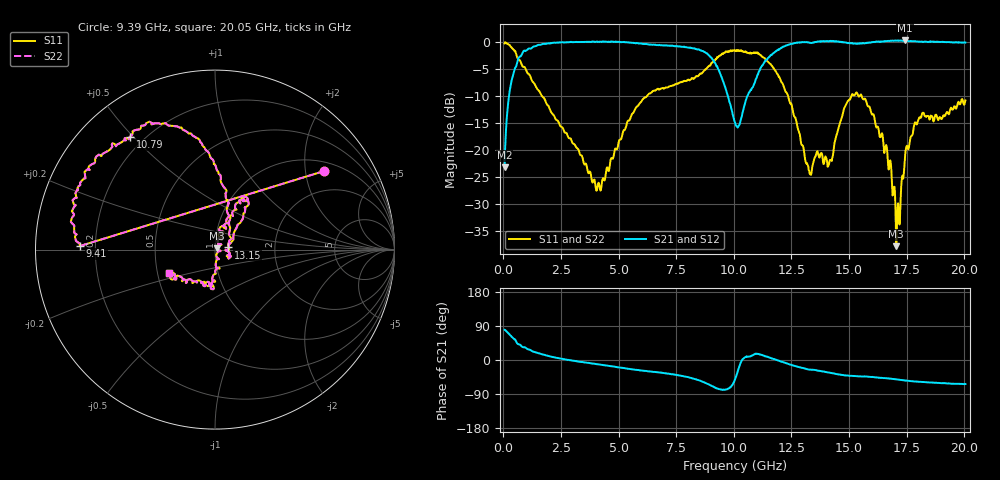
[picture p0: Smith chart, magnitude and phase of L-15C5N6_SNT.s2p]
#	mhz	s	ma	r	50
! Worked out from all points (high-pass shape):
!   1001 points, 50 MHz to 20.05 GHz, reference 50 ohm
!   highest |S21| = 0.31 dB at 17.43 GHz (marker M1); lowest = -23.2 dB at 50 MHz (marker M2)
!   |S21| within 3 dB of the highest: 708.4 MHz to 8.966 GHz (8.258 GHz wide, 171 % of centre); 11.54 GHz to end of sweep
!   lowest |S11| = -37.9 dB at 17.05 GHz (marker M3), VSWR 1.03, Z = 51.1 + j0.739 ohm
!   |S11| at or under -10 dB: 1.669 GHz to 6.236 GHz (4.567 GHz wide, 116 % of centre); 12.35 GHz to 15.1 GHz (2.748 GHz wide, 20 % of centre); 15.55 GHz to end of sweep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
!   |S22| runs from -37.9 to 0.0 dB; largest |S21 - S12| = 0
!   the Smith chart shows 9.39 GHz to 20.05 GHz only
!   S11 on the Smith chart (normalised r, x): 9.39 GHz: 1.27, +2.53; 9.41 GHz: 0.14, +0.01; 10.79 GHz: 0.15, +0.49; 13.15 GHz: 1.16, +0.03; 20.05 GHz: 0.58, -0.17
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50  0.9714 175.5  0.06904 79.7  0.06904 79.7  0.9714 175.5
310  0.9091 155.8  0.3928 64.5  0.3928 64.5  0.9091 155.8
750  0.6504 129.2  0.7373 38.7  0.7373 38.7  0.6504 129.2
1670  0.3159 100.5  0.9551 15.1  0.9551 15.1  0.3159 100.5
3390  0.08854 54.7  1.002 -5.3  1.002 -5.3  0.08854 54.7
4150  0.04844 -17.9  1.005 -11.7  1.005 -11.7  0.04844 -17.9
6730  0.3668 -115.6  0.9356 -32.7  0.9356 -32.7  0.3668 -115.6
8530  0.506 -143.6  0.8401 -54.4  0.8401 -54.4  0.506 -143.6
9390  0.7487 35.8  0.5203 -77.1  0.5203 -77.1  0.7487 35.8
9410  0.7527 178.5  0.5084 -77.5  0.5084 -77.5  0.7527 178.5
10050  0.839 153.7  0.1798 -51.3  0.1798 -51.3  0.839 153.7
10790  0.7869 126.9  0.3751 11.6  0.3751 11.6  0.7869 126.9
12070  0.4218 87.2  0.8868 -4.6  0.8868 -4.6  0.4218 87.2
13150  0.07446 9.2  1.001 -23.7  1.001 -23.7  0.07446 9.2
13390  0.06623 -3.5  0.9849 -25.5  0.9849 -25.5  0.06623 -3.5
14170  0.08047 6.2  1.02 -33.7  1.02 -33.7  0.08047 6.2
15250  0.3238 56.6  0.9695 -42.4  0.9695 -42.4  0.3238 56.6
16730  0.0656 57.0  1.027 -48.9  1.027 -48.9  0.0656 57.0
17050  0.01273 34.7  1.031 -51.1  1.031 -51.1  0.01273 34.7
17430  0.08663 -87.6  1.036 -53.9  1.036 -53.9  0.08663 -87.6
18150  0.2095 -96.4  1.012 -57.9  1.012 -57.9  0.2095 -96.4
20050  0.2875 -152.5  0.9908 -63.4  0.9908 -63.4  0.2875 -152.5
